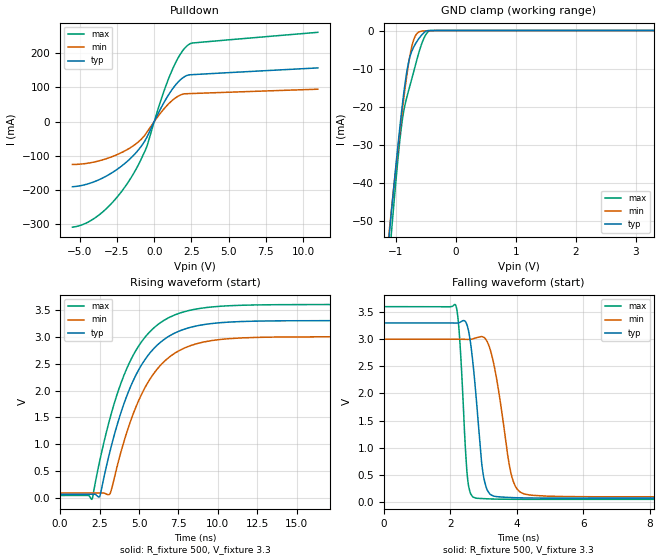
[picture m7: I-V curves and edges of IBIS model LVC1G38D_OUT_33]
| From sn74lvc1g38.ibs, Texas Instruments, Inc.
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[Model]   LVC1G38D_OUT_33
Model_type  Open_drain
Enable   Active-High
Vref =   3.3
Rref =   500
Cref =   50p
Vmeas =   1.5
| variable   typ   min   max
C_comp   3.82pF   2.94pF   5.06pF
| C_pulldown   7.20pF   4.59pF   11.10pF
| C_tri-state   3.82pF   2.94pF   5.06pF
[Temperature Range]   40   100   -40
| Ambient temperature   25   85   -40
[Voltage range]   3.3   3   3.6
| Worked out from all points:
|   slope of the pulldown table from 0 to 0.495 V, typ, clamps not added: 11.5 ohm
|   GND clamp passes 1 mA (typ) near -0.56 V on its own axis
|   rising waveform, R_fixture 500, V_fixture 3.3: 20-80 % time 2.54ns typ, 2.52ns min, 2.56ns max; typ from 0.07 V to 3.3 V
|   falling waveform, R_fixture 500, V_fixture 3.3: 20-80 % time 280ps typ, 429ps min, 183ps max; typ from 3.3 V to 0.07 V
[GND Clamp]
| LVC1G38D_OUT_33
|   Voltage   I(typ)   I(min)   I(max)
-5.5V     -916.4mA   -845.5mA   -1.045A
-1.13V    -57.53mA   -56.2mA    -64.35mA
-1.095V   -51.6mA    -50.76mA   -57.62mA
-1.065V   -46.59mA   -46.15mA   -51.95mA
-930mV    -25.31mA   -26.38mA   -28.72mA
-880mV    -18.33mA   -19.66mA   -22.49mA
-830mV    -12.35mA   -13.49mA   -18.5mA
-725mV    -5.18mA    -3.758mA   -12.29mA
-625mV    -2.368mA   -491.9uA   -6.381mA
-510mV    -327uA     -92.69uA   -1.403mA
-420mV    -4.422uA   -33.11uA   -10.75uA
3.3V      25.08pA    269.7pA    877.6pA
[Pulldown]
| LVC1G38D_OUT_33
|   Voltage   I(typ)   I(min)   I(max)
-5.5V     -190.2mA   -125.3mA   -308.2mA
-4.545V   -182.9mA   -122.1mA   -295.6mA
-3.555V   -166.5mA   -112.8mA   -267.1mA
-2.55V    -141.1mA   -97.46mA   -223.2mA
-1.61V    -108mA     -76.39mA   -167.4mA
-535mV    -49.07mA   -33.58mA   -76.9mA
455mV     39.78mA    26.61mA    63.54mA
1.16V     91.12mA    59.82mA    146mA
1.725V    120.6mA    76.78mA    194.8mA
2.245V    135.2mA    81.4mA     222.5mA
2.595V    137.1mA    81.95mA    229.5mA
11V       156.7mA    94.48mA    260.5mA
[Ramp]
| LVC1G38D_OUT_33
| variable   typ   min   max
dV/dt_r   1.97/2.55E-09   1.76/2.53E-09   2.17/2.57E-09
dV/dt_f   1.96/2.87E-10   1.77/4.44E-10   2.15/1.88E-10
R_load = 500
[Rising Waveform]
| LVC1G38D_OUT_33
R_fixture =   500
C_fixture =   0
L_fixture =   0
V_fixture =   3.3
V_fixture_min = 3
V_fixture_max = 3.6
|   Time   V(typ)   V(min)   V(max)
0s        70.47mV    94.51mV    48.4mV
2.02ns    70.49mV    94.5mV     -22.55mV
2.51ns    29.95mV    94.64mV    692.2mV
3.145ns   851.9mV    72.04mV    1.467V
4.025ns   1.738V     1.032V     2.268V
4.955ns   2.372V     1.798V     2.818V
5.89ns    2.765V     2.298V     3.151V
6.975ns   3.023V     2.634V     3.368V
10.87ns   3.275V     2.968V     3.579V
24.99ns   3.3V       3V         3.6V
[Falling Waveform]
| LVC1G38D_OUT_33
R_fixture =   500
C_fixture =   0
L_fixture =   0
V_fixture =   3.3
V_fixture_min = 3
V_fixture_max = 3.6
|   Time   V(typ)   V(min)   V(max)
0s        3.3V       3V         3.6V
2.16ns    3.298V     3V         3.632V
2.28ns    3.308V     2.999V     3.044V
2.52ns    3.232V     2.997V     443mV
2.77ns    1.998V     3.024V     70.34mV
2.955ns   670.6mV    3.048V     62.82mV
3.115ns   216.5mV    2.951V     58.16mV
3.845ns   80.98mV    484.8mV    49.41mV
4.28ns    74.31mV    139.7mV    48.68mV
24.99ns   70.47mV    94.51mV    48.4mV
